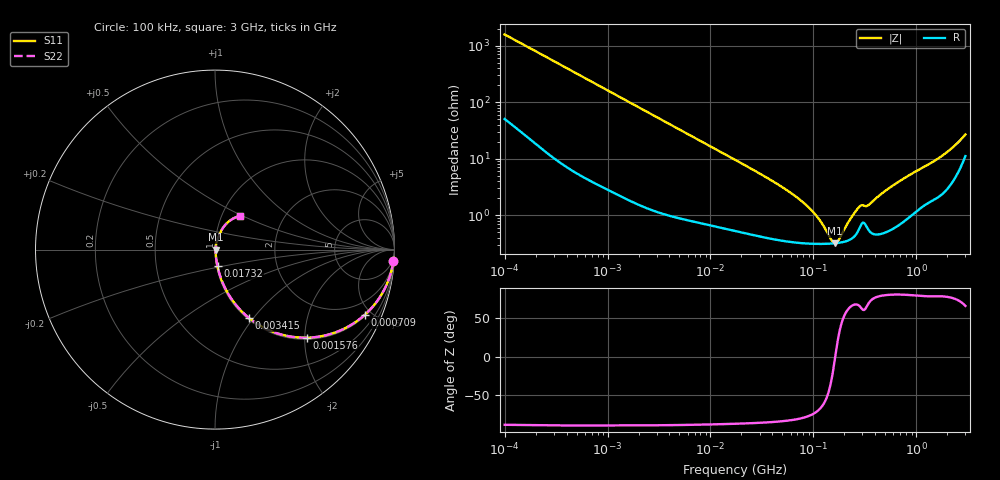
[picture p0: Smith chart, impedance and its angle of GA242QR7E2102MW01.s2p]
!Murata Part Number: GA242QR7E2102MW01
!These Parameters are Measured in Series Mode Connection
!Data Generated on Jun 19, 2026
!  o--ll--o
!Port1  Port2
!  o------o
!Operation Temp=25[degC], DC Bias Voltage=0[V]
!Freq. Start=100[kHz] Stop=3[GHz] 401[Steps]
# Hz S RI R 50
!Freq.(Hz) S11(Real) S11(Imag) S21(Real) S21(Imag) S12(Real) S12(Imag) S22(Real) S22(Imag)
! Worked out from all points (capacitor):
!   401 points, 100 kHz to 3 GHz, reference 50 ohm
!   read as one part in series: C = 1 nF near 105.3 kHz
!   lowest |Z| = 317 mohm at 163.1 MHz (marker M1)
!   series resonance near 163.1 MHz, so ESL is about 950 pH
!   S11 on the Smith chart (normalised r, x): 100 kHz: 2, -31; 709 kHz: 1.08, -4.54; 1.576 MHz: 1.04, -2.06; 3.415 MHz: 1.02, -0.96; 17.32 MHz: 1.01, -0.19; 3 GHz: 1.22, +0.49
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100000  0.994 -0.0629  0.006 0.0629  0.006 0.0629  0.994 -0.0629
246461  0.9738 -0.1497  0.0262 0.1497  0.0262 0.1497  0.9738 -0.1497
562235  0.8869 -0.3083  0.1131 0.3083  0.1131 0.3083  0.8869 -0.3083
709011  0.8335 -0.3641  0.1665 0.3641  0.1665 0.3641  0.8335 -0.3641
1576268  0.5141 -0.4908  0.4859 0.4908  0.4859 0.4908  0.5141 -0.4908
3161081  0.2151 -0.4003  0.7849 0.4003  0.7849 0.4003  0.2151 -0.4003
3415183  0.1911 -0.3823  0.8089 0.3823  0.8089 0.3823  0.1911 -0.3823
6674626  0.0633 -0.2283  0.9367 0.2283  0.9367 0.2283  0.0633 -0.2283
1.732051e7  0.014 -0.0934  0.986 0.0934  0.986 0.0934  0.014 -0.0934
1.77727e7  0.0136 -0.0911  0.9864 0.0911  0.9864 0.0911  0.0136 -0.0911
5.383243e7  0.00421 -0.0281  0.9958 0.0281  0.9958 0.0281  0.00421 -0.0281
9.738194e7  0.00322 -0.0113  0.9968 0.0113  0.9968 0.0113  0.00322 -0.0113
1.196798e8  0.00312 -0.00665  0.9969 0.00665  0.9969 0.00665  0.00312 -0.00665
1.509232e8  0.00312 -0.00166  0.9969 0.00166  0.9969 0.00166  0.00312 -0.00166
1.630551e8  0.00316 -1.01e-05  0.9968 1.01e-05  0.9968 1.01e-05  0.00316 -1.01e-05
1.761623e8  0.00321 0.00165  0.9968 -0.00165  0.9968 -0.00165  0.00321 0.00165
2.221509e8  0.00363 0.00691  0.9964 -0.00691  0.9964 -0.00691  0.00363 0.00691
2.730175e8  0.00541 0.0121  0.9946 -0.0121  0.9946 -0.0121  0.00541 0.0121
3.442911e8  0.00557 0.0139  0.9944 -0.0139  0.9944 -0.0139  0.00557 0.0139
5.475153e8  0.00611 0.0294  0.9939 -0.0294  0.9939 -0.0294  0.00611 0.0294
1.886474e9  0.0379 0.1108  0.9621 -0.1108  0.9621 -0.1108  0.0379 0.1108
3e9  0.1409 0.1881  0.8591 -0.1881  0.8591 -0.1881  0.1409 0.1881
